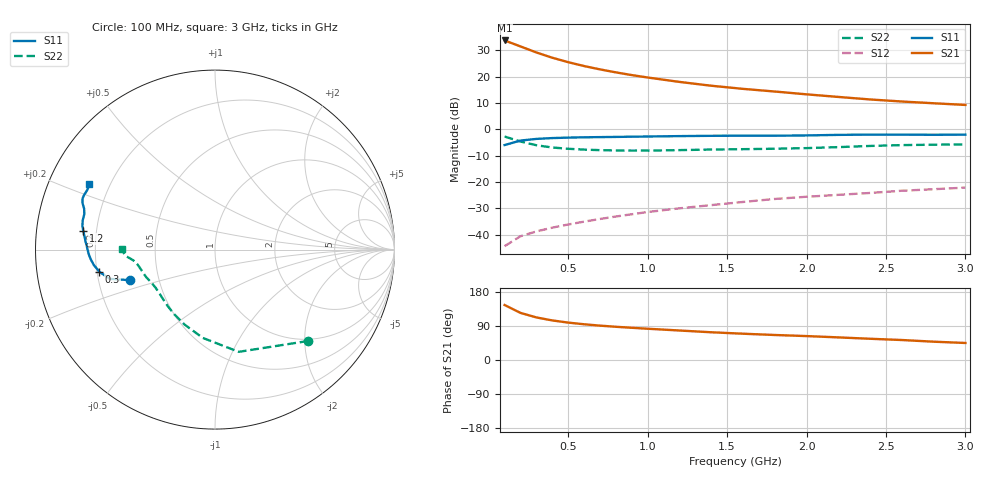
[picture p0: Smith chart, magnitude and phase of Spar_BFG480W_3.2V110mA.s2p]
! Filename: 3_2110BFG480.001
! Title: BFG480W
! Bias: Vce=3.2V; Ic=110mA
! Company: NXP Semiconductors NL
! User: Quality&Reliability T&D
! Measure time: 10 Nov 1999 / 11:58:12
#  MHz  S  MA  R 50
! Freq  S11  S21  S12  S22  :
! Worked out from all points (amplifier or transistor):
!   20 points, 100 MHz to 3 GHz, reference 50 ohm
!   highest |S21| = 33.7 dB at 100 MHz (marker M1)
!   |S21| within 3 dB of that: start of sweep to 231.8 MHz
!   unconditionally stable (mu >= 1): 640.3 MHz to end of sweep
!   at 400 MHz: K = 0.86, MSG = 32.3 dB, |S12| = -37.4 dB
!   at 1.2 GHz: K = 1.09, MAG = 22.2 dB, |S12| = -30.0 dB
!   at 3 GHz: K = 1.06, MAG = 14.2 dB, |S12| = -22.2 dB
!   S11 on the Smith chart (normalised r, x): 100 MHz: 0.34, -0.16; 300 MHz: 0.21, -0.09; 1.2 GHz: 0.15, +0.07; 3 GHz: 0.12, +0.24
100  0.5008 -160.1  48.64 145.1  0.006016 69.0  0.7276 -44.4
200  0.6098 -164.5  37.44 124.3  0.009296 61.3  0.5848 -76.9
300  0.6562 -169.2  28.77 112.3  0.01147 60.9  0.4968 -97.8
400  0.6802 -172.7  22.85 104.4  0.01353 62.9  0.4508 -112.1
500  0.6943 -175.5  18.82 98.7  0.01552 64.9  0.4258 -122.2
600  0.7035 -177.8  15.89 94.3  0.01757 66.8  0.411 -129.6
700  0.7097 -179.9  13.73 90.7  0.01977 68.9  0.4013 -135.4
800  0.7154 178.2  12.04 87.7  0.02201 70.4  0.3955 -140.1
900  0.7228 176.4  10.7 85.0  0.02428 72.0  0.393 -144.2
1000  0.7285 174.8  9.623 82.5  0.02679 72.9  0.3935 -147.8
1200  0.7412 171.9  7.936 77.8  0.03148 74.3  0.4016 -153.6
1400  0.7509 169.7  6.715 73.2  0.03622 75.0  0.4122 -157.9
1600  0.7548 167.4  5.857 69.4  0.0416 75.7  0.4187 -161.2
1800  0.7545 164.8  5.21 66.0  0.04743 75.9  0.4266 -164.8
2000  0.7636 162.7  4.61 63.1  0.05223 76.5  0.4385 -168.9
2200  0.7825 160.6  4.113 59.7  0.05676 76.3  0.4581 -172.4
2400  0.7911 158.9  3.683 56.0  0.0617 75.7  0.482 -174.6
2600  0.7901 157.2  3.367 52.7  0.06795 74.9  0.5002 -176.0
2800  0.785 154.9  3.12 48.3  0.07266 73.4  0.509 -177.8
3000  0.7905 152.2  2.897 44.9  0.07801 72.5  0.5168 179.4
